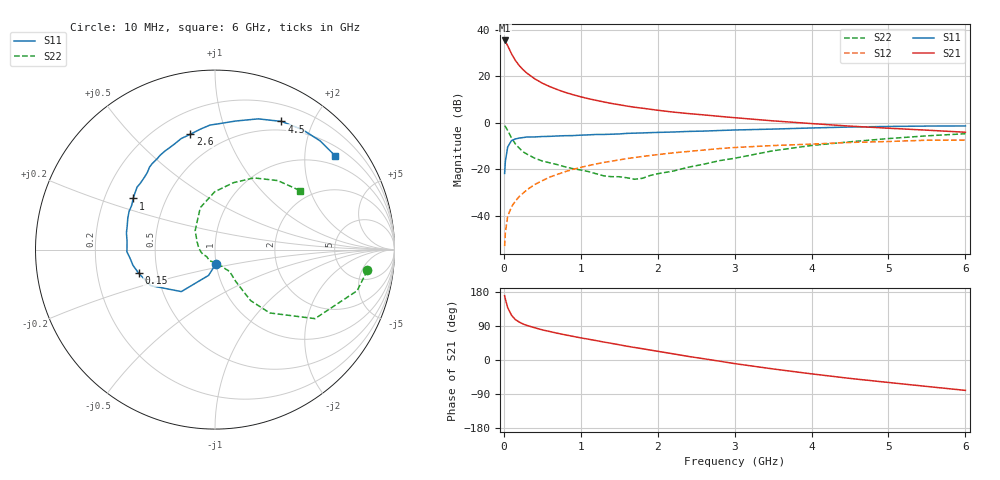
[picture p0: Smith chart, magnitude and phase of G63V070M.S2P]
! SIEMENS Small Signal Semiconductors
! BFG193
! Si NPN RF Bipolar Junction Transistor in SOT223
! VCE = 3 V  IC = 70 mA
! Common Emitter S-Parameters:  August  1996
# GHz  S  MA  R  50
!  f  S11  S21  S12  S22
! GHz  MAG  ANG  MAG  ANG  MAG  ANG  MAG  ANG
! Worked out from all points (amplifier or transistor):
!   36 points, 10 MHz to 6 GHz, reference 50 ohm
!   highest |S21| = 35.3 dB at 10 MHz (marker M1)
!   |S21| within 3 dB of that: start of sweep to 60.51 MHz
!   unconditionally stable (mu >= 1): start of sweep to 10.39 MHz; 302.9 MHz to 2.485 GHz
!   at 250 MHz: K = 0.99, MSG = 26.6 dB, |S12| = -30.3 dB
!   at 1.4 GHz: K = 1.06, MAG = 10.9 dB, |S12| = -16.6 dB
!   at 6 GHz: K = 0.92, MSG = 1.7 dB, |S12| = -7.5 dB
!   S11 on the Smith chart (normalised r, x): 10 MHz: 1.00, -0.16; 150 MHz: 0.39, -0.13; 1 GHz: 0.32, +0.26; 2.6 GHz: 0.33, +0.75; 4.5 GHz: 0.39, +1.58; 6 GHz: 0.73, +2.73
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0.01  0.0806 -86.5  58.54 169.7  0.0022 81.2  0.8563 -7.8
0.02  0.1481 -104.0  55.95 160.7  0.0043 83.5  0.8247 -16.1
0.05  0.2998 -128.7  45.06 138.1  0.0096 71.1  0.6772 -34.6
0.1  0.4112 -150.8  30.25 118.1  0.0155 69.0  0.4661 -49.2
0.15  0.4454 -162.9  21.72 106.5  0.0205 67.4  0.3474 -55.0
0.2  0.4651 -169.1  16.93 100.1  0.0257 70.0  0.2826 -55.8
0.25  0.4769 -174.6  13.76 95.0  0.0304 70.4  0.2356 -56.5
0.3  0.491 -178.6  11.6 91.2  0.0358 70.8  0.2105 -56.9
0.4  0.4919 174.8  8.797 85.2  0.0465 70.8  0.1721 -56.5
0.5  0.5022 169.2  7.054 79.5  0.0564 69.7  0.1494 -56.3
0.6  0.5069 164.7  5.927 75.0  0.0677 68.5  0.1362 -58.1
0.8  0.5238 156.1  4.462 66.3  0.0883 64.9  0.1113 -64.2
1  0.5377 148.0  3.589 58.4  0.109 61.4  0.0958 -71.9
1.1  0.5454 145.0  3.271 54.9  0.1187 59.5  0.0885 -79.6
1.3  0.5566 138.2  2.782 47.4  0.1394 55.4  0.0716 -93.0
1.6  0.5869 128.4  2.268 36.4  0.1683 48.3  0.0651 -124.4
2.2  0.6278 111.7  1.687 16.3  0.2234 34.4  0.0906 174.3
2.6  0.6575 102.0  1.466 3.3  0.2574 25.5  0.1277 145.1
3.5  0.7261 80.7  1.091 -23.6  0.3211 2.6  0.2482 109.2
4.5  0.8045 62.6  0.841 -48.6  0.3749 -17.7  0.3866 74.6
5.5  0.8426 46.0  0.688 -69.8  0.4186 -41.3  0.5199 47.7
6  0.8493 38.0  0.621 -80.2  0.4222 -54.7  0.5765 34.8
